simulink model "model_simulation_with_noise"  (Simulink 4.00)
settings: Solver=VariableStepDiscrete  StartTime=0.0  StopTime=ts  RelTol=1e-3
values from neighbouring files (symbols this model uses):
  A = [0.9944 -0.1203 -0.4302    [model_simple.m]
  Ao = A - K * C    [model_simple.m]
  B = [0.4252 -0.0082 0.1813]'    [model_simple.m]
  Bo = [B K]    [model_simple.m]
  C = [1 0 0]    [model_simple.m]
  Co = C    [model_simple.m]
  D = 0    [model_simple.m]
  Do = zeros(1,2)    [model_simple.m]
  Tc = 0.1    [model_simple.m]
  tfy = ts/2    (= 25)    [model_simple.m]
  x0 = [0.05 0.15 0.2]    [model_simple.m]

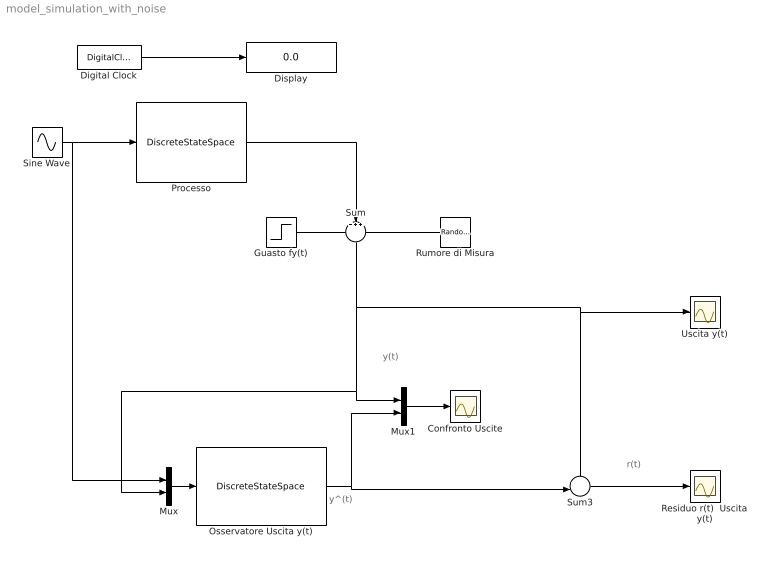
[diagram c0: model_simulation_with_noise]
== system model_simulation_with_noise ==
  note: y(t)
  note: y^(t)
  note: r(t)
  Confronto Uscite : Scope
  Digital Clock : DigitalClock  SampleTime=Tc
  Display : Display
  Guasto fy(t) : Step  Time=tfy  Before=0  After=1  SampleTime=Tc
  Mux : Mux  Inputs=2
  Mux1 : Mux  Inputs=2
  Osservatore Uscita y(t) : DiscreteStateSpace  A=Ao  B=Bo  C=Co  D=Do  X0=0  SampleTime=Tc  Realization=auto
  Processo : DiscreteStateSpace  A=A  B=B  C=C  D=D  X0=x0  SampleTime=Tc  Realization=auto
  Residuo r(t)  Uscita y(t) : Scope
  Rumore di Misura : RandomNumber  Orientation=left  Mean=0  Variance=0.05  Seed=0  SampleTime=Tc
  Sine Wave : Sin  SineType=Time-based  Amplitude=1  Bias=0  Frequency=1  Phase=0  Samples=10  SampleTime=Tc
  Sum : Sum  Orientation=down  Inputs=+++  SaturateOnIntegerOverflow=on
  Sum3 : Sum  Inputs=+-|  SaturateOnIntegerOverflow=on
  Uscita y(t) : Scope
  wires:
  Sine Wave/1 -> Processo/1, Mux/1
  Osservatore Uscita y(t)/1 -> Sum3/2, Mux1/2
  Mux/1 -> Osservatore Uscita y(t)/1
  Digital Clock/1 -> Display/1
  Sum3/1 -> Residuo r(t)  Uscita y(t)/1
  Mux1/1 -> Confronto Uscite/1
  Guasto fy(t)/1 -> Sum/1
  Processo/1 -> Sum/2
  Sum/1 -> Mux1/1, Mux/2, Sum3/1, Uscita y(t)/1
  Rumore di Misura/1 -> Sum/3
